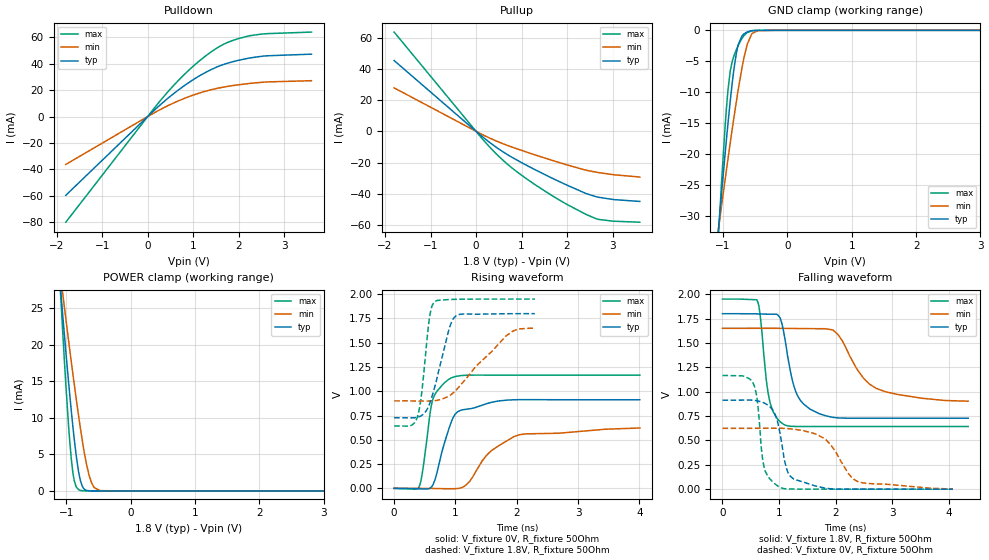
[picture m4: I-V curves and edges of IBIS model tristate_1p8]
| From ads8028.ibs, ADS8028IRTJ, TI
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|   tristate_1p8 Model
[Model]   tristate_1p8
Model_type   3-state
Polarity   Non-Inverting
Vmeas = 0.9
Vref = 0
Cref = 15pF
Rref = 150
|   typ   min   max
|   (nom PVT)   (fast PVT)   (slow PVT)
C_comp   1.328e-12   1.119e-12   1.577e-12
| Where nom  PVT is Nominal Process, 1.8V, 27C
|   Fast PVT is Strong Process,  1.95V, -40C
|   Slow PVT is Weak Process,   1.65V, 125C
[Voltage Range]   1.8   1.65   1.95
|Junction Temperature
[Temperature Range]   27   125   -40
[Pullup Reference]   1.8   1.65   1.95
[Pulldown Reference]   0   0   0
[Power Clamp Reference]   1.8   1.65   1.95
[GND Clamp Reference]   0   0   0
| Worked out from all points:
|   slope of the pulldown table from 0 to 0.27 V, typ, clamps not added: 31.2 ohm
|   slope of the pullup table from 0 to 0.27 V, typ, clamps not added: 41.8 ohm
|   GND clamp passes 1 mA (typ) near -0.71 V on its own axis
|   POWER clamp passes 1 mA (typ) near -0.77 V on its own axis
|   falling waveform, V_fixture 1.8V, R_fixture 50Ohm: 20-80 % time 254ps typ, 532ps min, 152ps max; typ from 1.8 V to 0.728 V
|   rising waveform, V_fixture 0V, R_fixture 50Ohm: 20-80 % time 256ps typ, 572ps min, 163ps max; typ from 0 V to 0.913 V
|   rising waveform, V_fixture 1.8V, R_fixture 50Ohm: 20-80 % time 258ps typ, 656ps min, 130ps max; typ from 0.728 V to 1.8 V
|   falling waveform, V_fixture 0V, R_fixture 50Ohm: 20-80 % time 198ps typ, 435ps min, 124ps max; typ from 0.913 V to 0 V
[Pulldown]
|   Voltage   I(typ)   I(min)   I(max)
-1.8V     -59.52mA   -36.21mA   -79.85mA
252mV     8.105mA    4.842mA    10.96mA
706.4mV   20.9mA     12.3mA     28.41mA
980.7mV   27.44mA    15.98mA    37.45mA
1.26V     33.11mA    19.03mA    45.45mA
1.525V    37.5mA     21.28mA    51.84mA
1.731V    40.06mA    22.63mA    55.63mA
1.979V    42.37mA    23.93mA    58.76mA
2.242V    44.26mA    25.04mA    61.09mA
2.642V    45.94mA    26.17mA    62.67mA
3.6V      47.14mA    27.09mA    63.82mA
[GND Clamp]
|   Voltage   I(typ)   I(min)   I(max)
-1.8V     -126.3mA   -91.94mA   -182.1mA
-1.084V   -33.59mA   -33.07mA   -35.53mA
-1.028V   -26.89mA   -28.71mA   -25.34mA
-945.9mV  -17.48mA   -22.46mA   -12.37mA
-891.3mV  -11.72mA   -18.41mA   -6.822mA
-828mV    -6.036mA   -13.88mA   -4.055mA
-768.4mV  -2.504mA   -9.874mA   -2.535mA
-709.4mV  -978.6uA   -6.266mA   -1.357mA
-625.2mV  -249.2uA   -2.271mA   -356.2uA
-554mV    -60.04uA   -564.1uA   -69.52uA
-458.6mV  -5.825uA   -53.34uA   -4.192uA
3.6V      0A         0A         0A
[Pullup]
|   Voltage   I(typ)   I(min)   I(max)
-1.8V     45.39mA    27.85mA    63.64mA
202.6mV   -4.928mA   -2.984mA   -6.976mA
511.2mV   -11.57mA   -7.011mA   -16.33mA
836.4mV   -17.43mA   -10.58mA   -24.56mA
1.283V    -24.4mA    -14.98mA   -33.92mA
1.764V    -31.32mA   -19.45mA   -42.88mA
2.41V     -39.79mA   -24.9mA    -53.18mA
2.65V     -42.03mA   -26.26mA   -56.17mA
3.003V    -43.69mA   -27.75mA   -57.6mA
3.6V      -44.98mA   -29.32mA   -58.28mA
[POWER Clamp]
|   Voltage   I(typ)   I(min)   I(max)
-1.8V     109mA      84.85mA    147.1mA
-1.105V   29.27mA    30.48mA    29.33mA
-1.063V   24.7mA     27.4mA     22.64mA
-1.028V   21.02mA    24.89mA    17.33mA
-963.5mV  14.63mA    20.38mA    8.577mA
-924.4mV  11.01mA    17.71mA    4.433mA
-874.8mV  6.827mA    14.39mA    1.296mA
-805.1mV  2.352mA    9.942mA    145.9uA
-734.1mV  358.2uA    5.879mA    12.84uA
-648mV    16.6uA     2.149mA    728.9nA
-478.3mV  40.49nA    41.84uA    0A
3.6V      0A         0A         0A
[Ramp]
R_load = 50
|   typ   min   max
dV/dt_r   0.54772/2.55445e-10   0.374476/5.76637e-10   0.699991/1.63055e-10
dV/dt_f   0.643339/2.53901e-10  0.449332/5.27335e-10   0.784372/1.50846e-10
[Falling Waveform]
V_fixture = 1.8V
V_fixture_min = 1.65V
V_fixture_max = 1.95V
R_fixture = 50Ohm
|   Time   V(typ)   V(min)   V(max)
0s        1.8V       1.65V      1.95V
614ps     1.798V     1.65V      1.936V
842ps     1.795V     1.65V      888.2mV
1.024ns   1.752V     1.65V      689.7mV
1.102ns   1.55V      1.649V     659.4mV
1.328ns   959.2mV    1.648V     642.8mV
1.71ns    774.7mV    1.646V     642.9mV
2.036ns   731.3mV    1.59V      642.8mV
2.724ns   728mV      1.033V     642.8mV
4.346ns   727.8mV    902.4mV    642.7mV
[Rising Waveform]
V_fixture = 0V
V_fixture_min = 0V
V_fixture_max = 0V
R_fixture = 50Ohm
|   Time   V(typ)   V(min)   V(max)
0s        950.5pV    8.614nV    779.9pV
402ps     -4.469mV   315.1uV    9.246mV
458ps     -5.718mV   223.2uV    151.1mV
584ps     1.474mV    -612.8uV   762.3mV
634ps     38.54mV    -1.133mV   922.3mV
926ps     672.8mV    -3.68mV    1.136V
1.076ns   802.3mV    2.573mV    1.161V
1.588ns   886.3mV    389mV      1.167V
2.038ns   913.7mV    551.1mV    1.166V
4.008ns   912.8mV    621.9mV    1.167V
[Rising Waveform]
V_fixture = 1.8V
V_fixture_min = 1.65V
V_fixture_max = 1.95V
R_fixture = 50Ohm
|   Time   V(typ)   V(min)   V(max)
0s        727.8mV    901.1mV    642.7mV
272ps     726.2mV    901.1mV    647.4mV
376ps     731.6mV    900.1mV    729.1mV
444ps     749mV      899.2mV    955.7mV
584ps     881mV      899.4mV    1.788V
660ps     1.038V     902.8mV    1.922V
894ps     1.638V     951.1mV    1.945V
1.008ns   1.776V     1.01V      1.947V
1.822ns   1.799V     1.568V     1.95V
2.296ns   1.8V       1.649V     1.95V
[Falling Waveform]
V_fixture = 0V
V_fixture_min = 0V
V_fixture_max = 0V
R_fixture = 50Ohm
|   Time   V(typ)   V(min)   V(max)
0s        912.9mV    624.1mV    1.167V
540ps     912.3mV    624.2mV    1.09V
614ps     906.1mV    624.3mV    919.4mV
748ps     881mV      624.8mV    199.3mV
1.018ns   571.5mV    624.8mV    19.53mV
1.132ns   215.5mV    622mV      3.541mV
1.262ns   103mV      615.3mV    1.34mV
1.818ns   10.67mV    514.1mV    156.8uV
2.406ns   533.6uV    73.75mV    80.2uV
4.074ns   31.71uV    1.326mV    4.865uV
